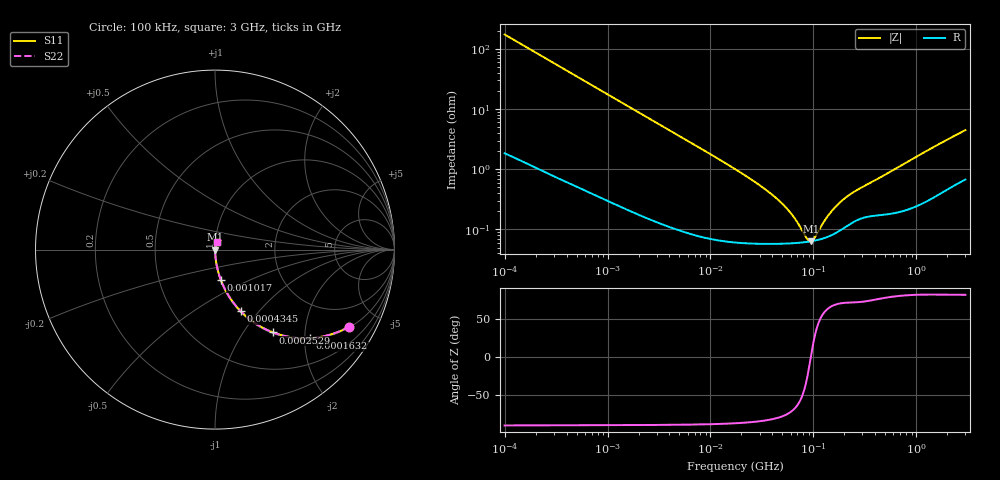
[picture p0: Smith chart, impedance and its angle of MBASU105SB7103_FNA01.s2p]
! MBASU105SB7103_FNA01  S-PARAMETER MODEL  ( Standard Model )
! Model Generated by TAIYO YUDEN Corporation (http://www.ty-top.com)
! Version 1.0
! TAIYO YUDEN Control No. 220601
! Copyright(c) 2013 TAIYO YUDEN CO.,LTD. All Rights Reserved.
! Product Description (link to TY-COMPAS)
! https://ds.yuden.co.jp/TYCOMPAS/or/detail?pn=MBASU105SB7103KFNA01&u=M
! Products Name : Multilayer Ceramic Capacitors
! Characteristics :
!  Capacitance : 0.01 [uF] , Rated Voltage : 50 [V] , TCC : X7R
!  Case Size : 1.0 x 0.5 / 0.039 x 0.02 [mm/inch] , Thickness : 0.5 / 0.02 [mm/inch]
!  (Conditions: Temperature = 25 [degC] , DC Bias Voltage = 0 [V])
! External Node Assignments :
!  1  o---| |---o  2
! GND o---------o GND
! Frequency Range : 100kHz  -  3GHz  [ 401 STEP ]
# MHZ S RI R 50
! Freq[MHz].  S11 Real  S11 Imag  S21 Real  S21 Imag  S12 Real  S12 Imag  S22 Real  S22 Imag
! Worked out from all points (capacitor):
!   401 points, 100 kHz to 3 GHz, reference 50 ohm
!   read as one part in series: C = 9.18 nF near 105.3 kHz
!   lowest |Z| = 63.7 mohm at 94.9 MHz (marker M1)
!   series resonance near 94.49 MHz, so ESL is about 310 pH
!   S11 on the Smith chart (normalised r, x): 100 kHz: 1.04, -3.46; 163.2 kHz: 1.03, -2.13; 252.9 kHz: 1.02, -1.38; 434.5 kHz: 1.01, -0.81; 1.017 MHz: 1.01, -0.35; 3 GHz: 1.01, +0.09
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0.1  0.7472 -0.4293  0.2528 0.4293  0.2528 0.4293  0.7472 -0.4293
0.163179  0.5306 -0.4932  0.4694 0.4932  0.4694 0.4932  0.5306 -0.4932
0.252895  0.3239 -0.4616  0.6761 0.4616  0.6761 0.4616  0.3239 -0.4616
0.4345  0.143 -0.3431  0.857 0.3431  0.857 0.3431  0.143 -0.3431
0.562235  0.0921 -0.2818  0.9079 0.2818  0.9079 0.2818  0.0921 -0.2818
1.017073  0.0319 -0.1673  0.9681 0.1673  0.9681 0.1673  0.0319 -0.1673
1.702975  0.0126 -0.1025  0.9874 0.1025  0.9874 0.1025  0.0126 -0.1025
3.161081  0.00443 -0.056  0.9956 0.056  0.9956 0.056  0.00443 -0.056
17.7727  0.0007 -0.00978  0.9993 0.00978  0.9993 0.00978  0.0007 -0.00978
32.15051  0.000601 -0.00496  0.9994 0.00496  0.9994 0.00496  0.000601 -0.00496
47.32384  0.000586 -0.00286  0.9994 0.00286  0.9994 0.00286  0.000586 -0.00286
64.47533  0.000594 -0.0015  0.9994 0.0015  0.9994 0.0015  0.000594 -0.0015
87.84301  0.000623 -0.000279  0.9994 0.000279  0.9994 0.000279  0.000623 -0.000279
94.90424  0.000636 1.71e-05  0.9994 -1.71e-05  0.9994 -1.71e-05  0.000636 1.71e-05
97.38194  0.000641 0.000116  0.9994 -0.000116  0.9994 -0.000116  0.000641 0.000116
105.21  0.000658 0.000413  0.9993 -0.000413  0.9993 -0.000413  0.000658 0.000413
139.694  0.000764 0.00154  0.9992 -0.00154  0.9992 -0.00154  0.000764 0.00154
190.323  0.00102 0.00285  0.999 -0.00285  0.999 -0.00285  0.00102 0.00285
259.3015  0.00141 0.00418  0.9986 -0.00418  0.9986 -0.00418  0.00141 0.00418
547.5153  0.00188 0.00869  0.9981 -0.00869  0.9981 -0.00869  0.00188 0.00869
1535  0.00408 0.0239  0.9959 -0.0239  0.9959 -0.0239  0.00408 0.0239
3000  0.00859 0.0434  0.9914 -0.0434  0.9914 -0.0434  0.00859 0.0434
